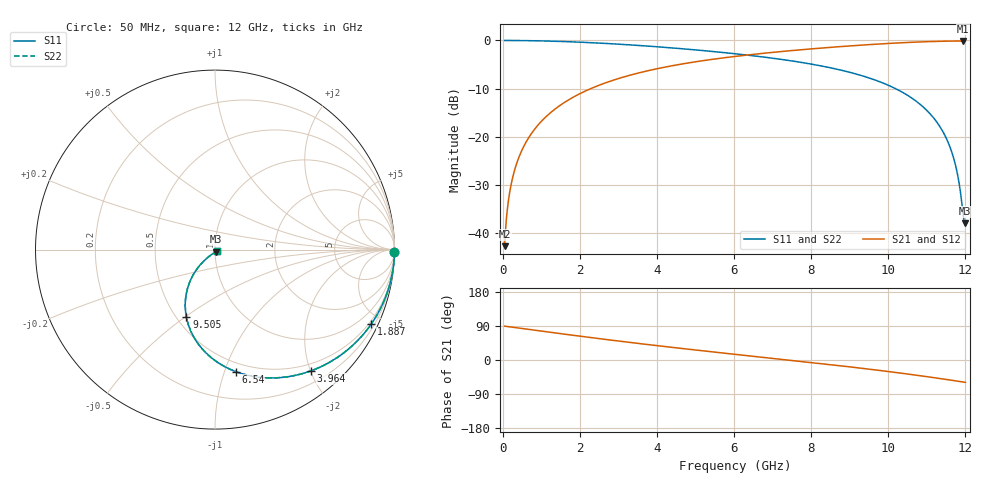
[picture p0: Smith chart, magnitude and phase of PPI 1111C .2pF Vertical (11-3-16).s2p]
# GHz S MA R 50
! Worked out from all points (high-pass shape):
!   1601 points, 50 MHz to 12 GHz, reference 50 ohm
!   highest |S21| = -0.11 dB at 11.93 GHz (marker M1); lowest = -42.8 dB at 50 MHz (marker M2)
!   |S21| within 3 dB of the highest: 6.247 GHz to end of sweep
!   lowest |S11| = -38.0 dB at 11.99 GHz (marker M3), VSWR 1.03, Z = 50.6 - j1.11 ohm
!   |S11| at or under -10 dB: 10.18 GHz to end of sweep
!   |S22| runs from -38.0 to 0.0 dB; largest |S21 - S12| = 0
!   S11 on the Smith chart (normalised r, x): 50 MHz: open; 1.887 GHz: 0.37, -4.38; 3.964 GHz: 0.38, -2.01; 6.54 GHz: 0.42, -1.09; 9.505 GHz: 0.56, -0.50; 12 GHz: 1.02, -0.02
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0.05  1 -0.7  0.007258 89.3  0.007258 89.3  1 -0.7
0.1545625  0.9997 -2.1  0.02243 87.9  0.02243 87.9  0.9997 -2.1
0.2367188  0.9994 -3.3  0.03434 86.7  0.03434 86.7  0.9994 -3.3
0.3711563  0.9985 -5.1  0.0538 84.9  0.0538 84.9  0.9985 -5.1
0.5429375  0.9969 -7.5  0.07858 82.5  0.07858 82.5  0.9969 -7.5
1.080688  0.9878 -14.8  0.155 75.2  0.155 75.2  0.9878 -14.8
1.887312  0.964 -25.6  0.2647 64.4  0.2647 64.4  0.964 -25.6
2.044156  0.9582 -27.6  0.285 62.3  0.285 62.3  0.9582 -27.6
3.963625  0.8622 -51.5  0.5043 38.4  0.5043 38.4  0.8622 -51.5
4.038312  0.8578 -52.4  0.5117 37.5  0.5117 37.5  0.8578 -52.4
6.025  0.7276 -74.8  0.6821 15.0  0.6821 15.0  0.7276 -74.8
6.540344  0.6896 -80.3  0.7198 9.3  0.7198 9.3  0.6896 -80.3
8.019156  0.5663 -96.3  0.8182 -6.9  0.8182 -6.9  0.5663 -96.3
9.505437  0.4071 -113.1  0.9053 -24.2  0.9053 -24.2  0.4071 -113.1
10.01331  0.3404 -119.1  0.9313 -30.5  0.9313 -30.5  0.3404 -119.1
10.82741  0.2165 -128.8  0.9657 -41.5  0.9657 -41.5  0.2165 -128.8
11.38009  0.1194 -134.1  0.9811 -49.5  0.9811 -49.5  0.1194 -134.1
11.71619  0.0558 -132.2  0.986 -54.6  0.986 -54.6  0.0558 -132.2
11.82075  0.03584 -126.3  0.9866 -56.2  0.9866 -56.2  0.03584 -126.3
11.93278  0.01664 -99.5  0.9869 -58.0  0.9869 -58.0  0.01664 -99.5
11.98506  0.01259 -60.2  0.9868 -58.8  0.9868 -58.8  0.01259 -60.2
12  0.01291 -46.7  0.9868 -59.0  0.9868 -59.0  0.01291 -46.7
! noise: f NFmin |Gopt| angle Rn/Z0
0.05  0.00371  0.9928  0.6844  0.1177
1.372  0.006336  0.8413  13.21  0.008355
2.701  0.009334  0.7663  20.56  0.007869
4.031  0.01227  0.7285  26.86  0.008521
5.36  0.01522  0.7094  32.8  0.00951
6.682  0.01827  0.7018  38.45  0.01074
8.012  0.02156  0.7026  43.89  0.01228
9.341  0.02518  0.7098  49.09  0.01422
10.67  0.02928  0.7224  54.07  0.0167
12  0.03405  0.7393  58.86  0.01998
